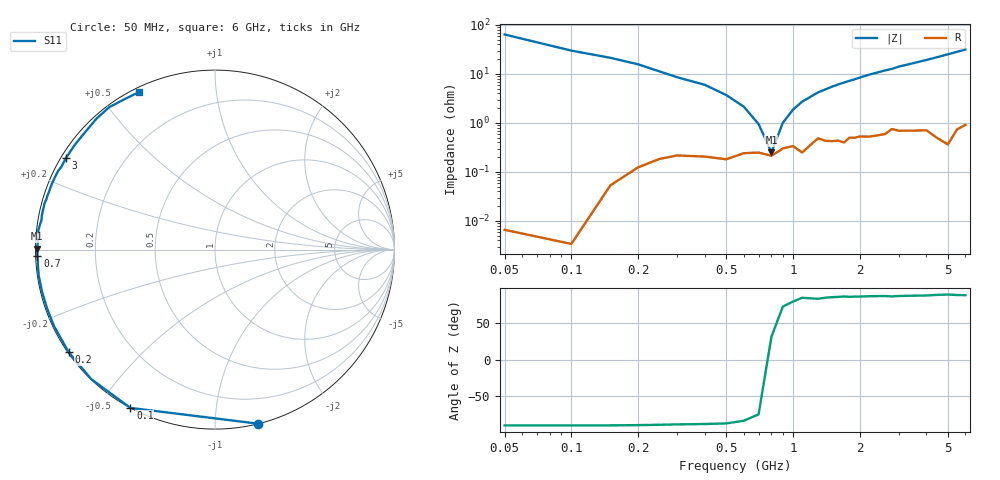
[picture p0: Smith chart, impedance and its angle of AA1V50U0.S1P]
! Infineon Technologies  Discrete & RF Semiconductors
! BBY66-02W
! Si Tuning Diode in SCD-80
! VR = 1.5 V
! S-Parameters:  June  2000
# GHz  S  MA  R  50
!  f  S11
! GHz  MAG  ANG
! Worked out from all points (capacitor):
!   34 points, 50 MHz to 6 GHz, reference 50 ohm
!   read as one part to ground: C = 49.5 pF near 50 MHz
!   lowest |Z| = 250 mohm at 800 MHz (marker M1)
!   series resonance near 787.5 MHz, so ESL is about 820 pH
!   S11 on the Smith chart (normalised r, x): 50 MHz: 0.00, -1.28; 100 MHz: 0.00, -0.60; 200 MHz: 0.00, -0.32; 700 MHz: 0.00, -0.02; 3 GHz: 0.01, +0.28; 6 GHz: 0.02, +0.63
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0.05  0.9999 -76.0
0.1  0.9999 -118.1
0.15  0.9982 -133.7
0.2  0.9955 -145.0
0.25  0.993 -154.6
0.3  0.9916 -160.5
0.4  0.9919 -166.3
0.5  0.9928 -171.5
0.6  0.9904 -175.1
0.7  0.9901 -177.9
0.8  0.9915 179.7
1  0.9866 175.8
1.1  0.9901 173.8
1.3  0.9808 170.4
1.6  0.983 166.1
1.7  0.9844 164.8
1.9  0.9807 162.3
2.2  0.9799 158.2
2.4  0.9789 155.9
2.6  0.9778 153.5
2.8  0.9721 151.5
3  0.9746 148.5
3.5  0.9752 143.2
4  0.9756 137.8
4.5  0.9839 132.2
5  0.9884 126.6
5.5  0.9779 120.9
6  0.9742 115.6
